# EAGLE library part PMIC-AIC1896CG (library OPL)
1. 4MHz Thin Package Current-Mode Step-Up DC/DC Converter
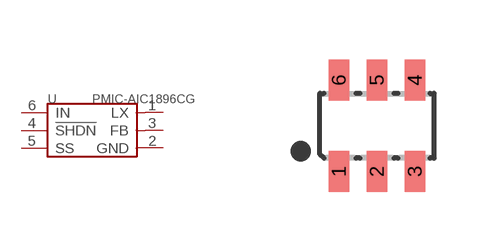
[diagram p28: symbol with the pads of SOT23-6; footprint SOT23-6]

Designator prefix U

## PMIC-AIC1896CG-310030104  [SOT23-6]
1  LX  out
2  GND  pwr
3  FB  in
4  !SHDN  in
5  SS  in
6  IN  in

## Footprint SOT23-6 (pad centres in mm)
smd 0.508 x 1.016: 1 -0.95,-1.143; 2 0,-1.143; 3 0.95,-1.143; 4 0.95,1.143; 5 0,1.143; 6 -0.95,1.143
